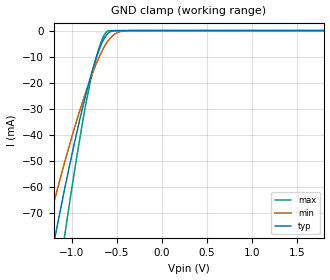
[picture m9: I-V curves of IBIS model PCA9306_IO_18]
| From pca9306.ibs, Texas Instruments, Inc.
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[Model]   PCA9306_IO_18
Model_type  Terminator
| variable   typ   min   max
C_comp   2.75pF   2.40pF   3.22pF
| C_tri-state   2.75pF   2.40pF   3.22pF
[Temperature Range]   40   100   -40
| Ambient temperature   25   85   -40
[Voltage range]   1.8   1.65   1.95
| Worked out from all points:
|   GND clamp passes 1 mA (typ) near -0.59 V on its own axis
[GND Clamp]
| PCA9306_IO_18
|   Voltage   I(typ)   I(min)   I(max)
-1.8V     -199mA     -155.3mA   -267.3mA
-1.285V   -97.6mA    -78.12mA   -129.7mA
-1.18V    -78.63mA   -63.89mA   -103.5mA
-1.16V    -75.11mA   -61.25mA   -98.65mA
-1.08V    -61.36mA   -50.98mA   -79.54mA
-1.06V    -58.02mA   -48.48mA   -74.88mA
-900mV    -32.89mA   -29.77mA   -39.72mA
-785mV    -17.27mA   -18.04mA   -18.52mA
-680mV    -6.109mA   -9.157mA   -5.225mA
-600mV    -1.21mA    -4.203mA   -179.9uA
-380mV    -1.17uA    -64.95uA   -13.15nA
1.8V      22.1pA     2.885nA    8.051pA
